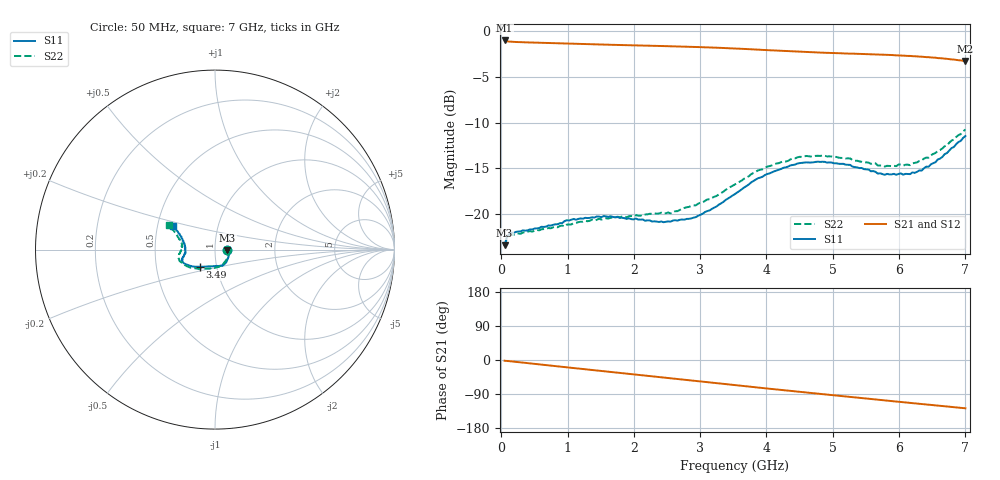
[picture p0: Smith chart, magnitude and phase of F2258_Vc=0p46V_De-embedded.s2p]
! Integrated Device Technology
! Corporate Headquarters
! 6024 Silver Creek Valley Road
! San Jose, CA 95138  USA
! Phone:  1-408-284-8200
! Toll Free:  1-800-223-1366
! Webpage:  http://www.idt.com/
! Timing and RF Division
! 515 Groton Road, Suite 102
! Westford, MA 01886-6024
! Device:  F2258
! Description: Voltage Variable RF Attenuator
! Frequency:  50.0 -  6000.00 MHz
! Package:  3x3 mm Thin QFN Plastic Package: 16 pin
! Ports:  2 RF, 2 DC
!  Pin  1  = NC
!  Pin  2  = NC
!  Pin  3  = RF2  = Port 2
!  Pin  4  = GND
!  Pin  5  = Vdd
!  Pin  6  = NC
!  Pin  7  = VCTRL
!  Pin  8  = NC
!  Pin  9  = GND
!  Pin 10  = RF1  = Port 1
!  Pin 11  = NC
!  Pin 12  = NC
!  Pin 13  = NC
!  Pin 14  = NC
!  Pin 15  = NC
!  Pin 16  = NC
! Vcntrl:  0.460 Volts
! Vdd:  +3.300 Volts
! Current:  1.095 mA
! Data:  The device was measured on a the F2258 evaluation board which has
!  individual transmission lines to the RF pins.  Data was collected
!  using a calibrated network analyzer.  The evaluation board was
!  de-embedded using a TRL calibration technique.
!  The reference plane is the edge of the package pin.
! Misc:  SN 10
!  Action Tracker AT0285
! Date Measured:  2014-12-10
! Date:  2016-01-13  MJV
! Note:
!  Integrated Device Technology supplies this data as a sample of measured
!  data at the package pin for this product.  Your particular data for this
!  product may vary.
!  Data was taken at 25 degrees C.
!  Integrated Device Technology reserves the right to change this data at anytime.
!Freq_(GHz)  S11M_(dB)  S11P_(deg)  S21M_(dB)  S21P_(deg)  S12M_(dB)  S12P_(deg)  S22M_(dB)  S22P_(deg)
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# GHz S dB R 50
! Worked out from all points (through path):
!   201 points, 50 MHz to 7 GHz, reference 50 ohm
!   highest |S21| = -1.06 dB at 50 MHz (marker M1); lowest = -3.3 dB at 7 GHz (marker M2)
!   group delay of S21, straight-line fit = 50.5 ps
!   lowest |S11| = -23.4 dB at 50 MHz (marker M3), VSWR 1.15, Z = 57.3 - j0.441 ohm
!   |S11| at or under -10 dB: start of sweep to end of sweep
!   |S22| runs from -23.5 to -10.8 dB; largest |S21 - S12| = 0.00047
!   S11 on the Smith chart (normalised r, x): 50 MHz: 1.15, -0.01; 3.49 GHz: 0.83, -0.16; 7 GHz: 0.61, +0.17
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0.05  -23.36 -3.2  -1.06 -2.0  -1.06 -2.0  -23.46 -3.1
0.08475  -22.44 -5.2  -1.15 -2.5  -1.15 -2.5  -22.57 -5.1
0.15425  -21.98 -8.1  -1.20 -3.7  -1.20 -3.7  -22.20 -8.8
0.71025  -21.20 -33.2  -1.34 -14.1  -1.34 -14.1  -21.48 -36.2
1.2315  -20.46 -54.0  -1.45 -23.8  -1.45 -23.8  -20.79 -60.3
1.6485  -20.19 -65.2  -1.53 -31.4  -1.53 -31.4  -20.36 -73.4
2.37825  -20.82 -85.2  -1.66 -44.8  -1.66 -44.8  -19.90 -91.7
2.552  -20.79 -91.0  -1.69 -48.0  -1.69 -48.0  -19.89 -97.0
2.93425  -20.30 -107.7  -1.77 -55.1  -1.77 -55.1  -19.01 -110.6
3.247  -19.13 -121.0  -1.85 -61.0  -1.85 -61.0  -18.00 -122.9
3.49025  -17.93 -131.3  -1.93 -65.6  -1.92 -65.6  -16.87 -132.2
3.525  -17.78 -132.3  -1.94 -66.2  -1.94 -66.2  -16.74 -133.7
4.0115  -15.60 -147.2  -2.12 -75.3  -2.12 -75.3  -14.79 -149.5
4.46325  -14.47 -156.1  -2.28 -83.4  -2.28 -83.4  -13.79 -160.8
4.7065  -14.33 -159.5  -2.35 -87.7  -2.35 -87.7  -13.68 -165.1
5.2625  -14.61 -166.2  -2.50 -97.4  -2.50 -97.4  -13.91 -173.4
5.6795  -15.56 -172.6  -2.59 -104.6  -2.59 -104.6  -14.68 -179.0
5.85325  -15.64 -176.8  -2.64 -107.8  -2.64 -107.8  -14.72 176.4
6.166  -15.61 175.2  -2.75 -113.4  -2.75 -113.3  -14.64 170.3
6.33975  -15.23 168.6  -2.83 -116.5  -2.83 -116.5  -14.13 165.9
6.722  -13.32 156.0  -3.06 -123.1  -3.06 -123.1  -12.49 156.7
7  -11.47 150.1  -3.31 -127.4  -3.31 -127.4  -10.76 151.7
